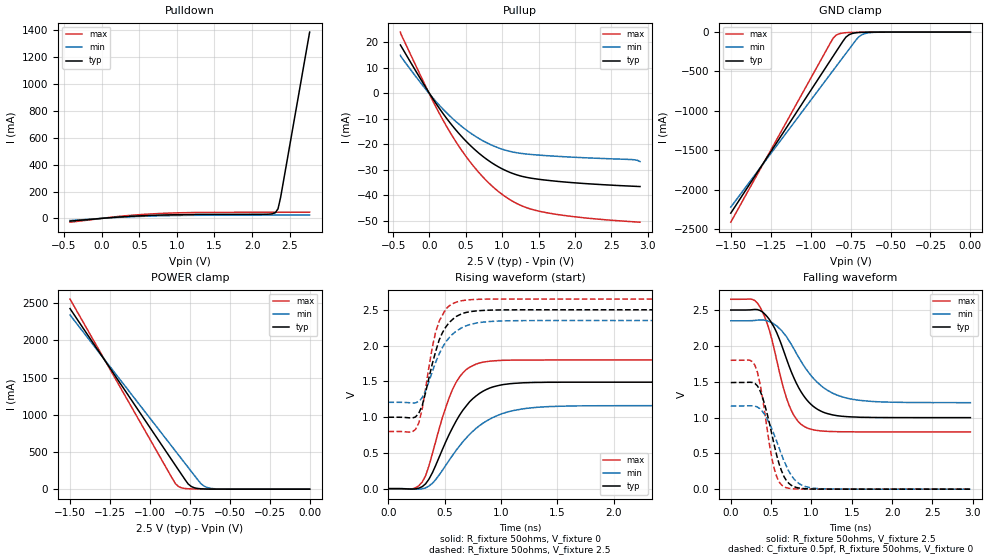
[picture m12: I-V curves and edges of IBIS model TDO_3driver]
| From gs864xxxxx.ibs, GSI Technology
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|  signals   TDO
[Model]   TDO_3driver
Model_type   3-state
Polarity   Non-Inverting
Vmeas =   1.25v
Cref  =   0pF
Rref  =   50
Vref  =   1.25v
|  variable   typ   min   max
C_comp   3.0pF   2.5pF   3.5pF
|  variable   typ   min   max
[Temperature Range]   50   0   100
|  variable   typ   min   max
[Voltage Range]   2.5   2.35   2.65
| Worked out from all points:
|   slope of the pulldown table from 0 to 0.375 V, typ, clamps not added: 24.9 ohm
|   slope of the pullup table from 0 to 0.375 V, typ, clamps not added: 25.4 ohm
|   GND clamp passes 1 mA (typ) near -0.63 V on its own axis
|   POWER clamp passes 1 mA (typ) near -0.62 V on its own axis
|   rising waveform, R_fixture 50ohms, V_fixture 0: 20-80 % time 297ps typ, 384ps min, 219ps max; typ from 0 V to 1.49 V
|   rising waveform, R_fixture 50ohms, V_fixture 2.5: 20-80 % time 164ps typ, 201ps min, 132ps max; typ from 0.998 V to 2.5 V
|   falling waveform, R_fixture 50ohms, V_fixture 2.5: 20-80 % time 344ps typ, 434ps min, 263ps max; typ from 2.5 V to 0.998 V
|   falling waveform, C_fixture 0.5pf, R_fixture 50ohms, V_fixture 0: 20-80 % time 198ps typ, 256ps min, 156ps max; typ from 1.49 V to 0 V
[Pulldown]
| voltage   I(typ)   I(min)   I(max)
-420mV    -20.34mA   -15.77mA   -28.32mA
245mV     10.63mA    8.095mA    15.57mA
735mV     23.82mA    18.55mA    35.34mA
1.19V     28.64mA    22.79mA    43.21mA
2.205V    30.99mA    24.48mA    45.48mA
2.275V    34.57mA    24.53mA    45.55mA
2.31V     43.04mA    24.56mA    45.59mA
2.345V    71.54mA    24.58mA    45.62mA
2.38V     158.7mA    24.61mA    45.65mA
2.765V    1.386A     24.87mA    45.99mA
[Pullup]
| voltage (VDDQ-Vout) I(typ)   I(min)   I(max)
-400mV    19.02mA    14.94mA    24.06mA
25mV      -1.125mA   -1.034mA   -1.743mA
305mV     -12.33mA   -9.521mA   -16.29mA
480mV     -18.07mA   -13.78mA   -23.84mA
620mV     -21.97mA   -16.62mA   -29.05mA
760mV     -25.28mA   -18.97mA   -33.55mA
935mV     -28.6mA    -21.23mA   -38.19mA
1.215V    -32.08mA   -23.35mA   -43.4mA
1.495V    -33.66mA   -24.18mA   -46.13mA
2.125V    -35.34mA   -25.23mA   -48.8mA
2.79V     -36.4mA    -25.97mA   -50.33mA
2.895V    -36.53mA   -26.74mA   -50.52mA
[GND Clamp]
| voltage   I(typ)   I(min)   I(max)
-1.5V     -2.3A      -2.224A    -2.415A
-880mV    -370.6mA   -543.1mA   -151.1mA
-860mV    -308.5mA   -489mA     -80.12mA
-840mV    -246.5mA   -434.9mA   -38.91mA
-820mV    -184.4mA   -380.9mA   -20.22mA
-780mV    -65.55mA   -272.8mA   -7.662mA
-760mV    -33.81mA   -218.9mA   -5.572mA
-700mV    -5.364mA   -62.59mA   -2.825mA
-660mV    -1.94mA    -18.77mA   -1.788mA
-560mV    -225.3uA   -949.8uA   -330.3uA
0V        -98.92pA   -343.3pA   -54.9pA
[POWER Clamp]
| voltage (VDDQ-Vout) I(typ)   I(min)   I(max)
-1.5V     2.426A     2.341A     2.554A
-860mV    382.9mA    567.6mA    145.1mA
-840mV    319.2mA    512.3mA    73.64mA
-820mV    255.5mA    457.1mA    33.99mA
-800mV    191.9mA    401.8mA    16.54mA
-760mV    68.92mA    291.3mA    5.271mA
-740mV    34.64mA    236.1mA    3.556mA
-680mV    4.879mA    73.28mA    1.644mA
-640mV    1.574mA    21.56mA    1.043mA
-540mV    157.9uA    1.034mA    211.3uA
0V        141.2pA    565.8pA    59.03pA
[Ramp]
| voltage   typ   min   max
dV/dt_r   0.89/220p   0.71/258p   1.11/185p
dV/dt_f   1.05/247p   0.91/322p   1.22/196p
R_load  =   50ohms
[Rising Waveform]
C_fixture =   0.0pf
R_fixture =   50ohms
V_fixture =   0
| Time   V(typ)   V(min)   V(max)
0s        1.363nV    5.964nV    579.4pV
210ps     -6.138mV   -5.067mV   -3.188mV
300ps     28.16mV    -2.394mV   91.34mV
390ps     220.6mV    74.09mV    487mV
570ps     853.5mV    466.7mV    1.389V
660ps     1.094V     653.6mV    1.616V
780ps     1.298V     845.5mV    1.742V
1.02ns    1.455V     1.054V     1.794V
1.29ns    1.484V     1.133V     1.798V
2.97ns    1.488V     1.16V      1.799V
[Rising Waveform]
C_fixture =   0.0pf
R_fixture =   50ohms
V_fixture =   2.5
V_fixture_min =   2.35
V_fixture_max =   2.65
| Time   V(typ)   V(min)   V(max)
0s        998.1mV    1.207V     799mV
240ps     1.001V     1.199V     827.3mV
270ps     1.055V     1.218V     918.4mV
300ps     1.162V     1.272V     1.112V
390ps     1.748V     1.636V     1.978V
420ps     1.92V      1.769V     2.194V
510ps     2.261V     2.052V     2.513V
600ps     2.405V     2.199V     2.606V
990ps     2.498V     2.343V     2.65V
2.97ns    2.5V       2.35V      2.65V
[Falling Waveform]
C_fixture =   0.0pf
R_fixture =   50ohms
V_fixture =   2.5
V_fixture_min =   2.35
V_fixture_max =   2.65
| Time   V(typ)   V(min)   V(max)
0s        2.5V       2.35V      2.65V
270ps     2.505V     2.352V     2.647V
360ps     2.495V     2.362V     2.547V
450ps     2.409V     2.351V     2.317V
540ps     2.254V     2.301V     1.946V
720ps     1.726V     2.075V     1.179V
930ps     1.263V     1.682V     863.1mV
1.17ns    1.064V     1.401V     808.4mV
1.5ns     1.008V     1.256V     800.1mV
2.97ns    998.2mV    1.207V     799mV
[Falling Waveform]
C_fixture =   0.5pf
R_fixture =   50ohms
V_fixture =   0
| Time   V(typ)   V(min)   V(max)
0s        1.488V     1.16V      1.799V
300ps     1.475V     1.159V     1.728V
390ps     1.295V     1.087V     1.3V
480ps     917.5mV    913.1mV    621.8mV
540ps     609.2mV    753.7mV    280.4mV
600ps     349.2mV    571.2mV    99.15mV
660ps     175.4mV    393.4mV    34.15mV
810ps     25.07mV    109.6mV    3.273mV
1.02ns    2.269mV    14.49mV    290uV
2.97ns    443.9nV    1.056uV    216nV
